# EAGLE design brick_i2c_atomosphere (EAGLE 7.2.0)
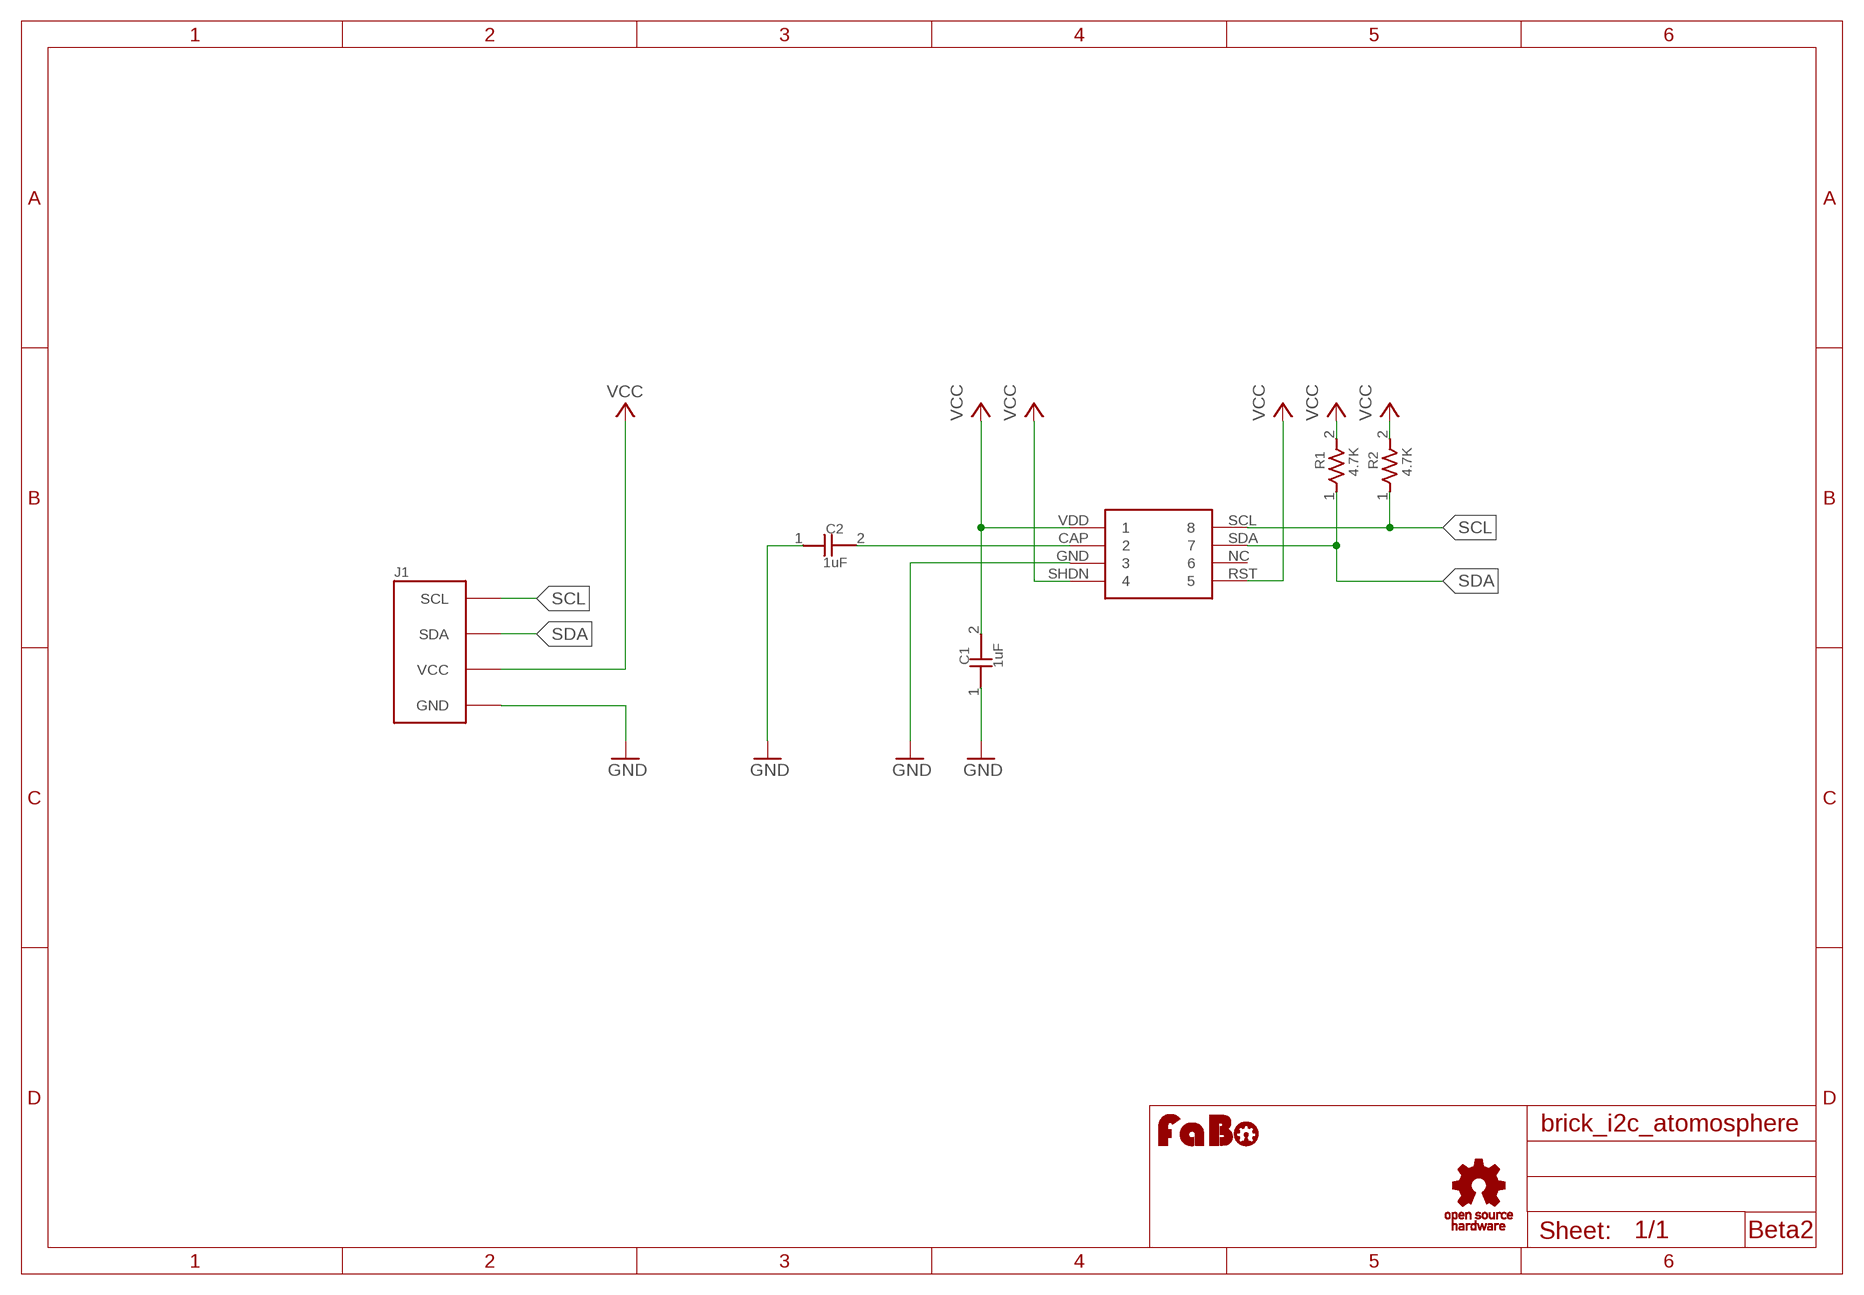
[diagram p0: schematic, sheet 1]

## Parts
C1  1uF  CAPACITOR0603  [0603]
C2  1uF  CAPACITOR0603  [0603]
J1  BRICK_I2C  [BRICK_I2C]
R1  4.7K  RESISTOR0603  [0603]
R2  4.7K  RESISTOR0603  [0603]
U$2  I2C-MPL115A2  [I2C-MLP115A2]
U$3  LOGO_FABO-M  [LOGO_FABO_M]
U$5  LOGO_OSHW_T-M  [LOGO_OSHW_T_M]

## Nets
GND: C1.1 C2.1 J1.GND U$2.GND
N$1: C2.2 U$2.CAP
SCL: J1.SCL R2.1 U$2.SCL
SDA: J1.SDA R1.1 U$2.SDA
VCC: C1.2 J1.VCC R1.2 R2.2 U$2.RST U$2.SHDN U$2.VDD
Unconnected: U$2.NC

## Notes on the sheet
- Beta2

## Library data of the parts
C1 C2 = GClue-Capacitor:CAPACITOR
J1 = gclue:BRICK_I2C: FaBo Brick 4pin(I2C)
R1 R2 = GClue-Resistors:RESISTOR
U$2 = gclue:I2C-MPL115A2
U$3 = FaBo:LOGO_FABO
U$5 = gclue:LOGO_OSHW_T

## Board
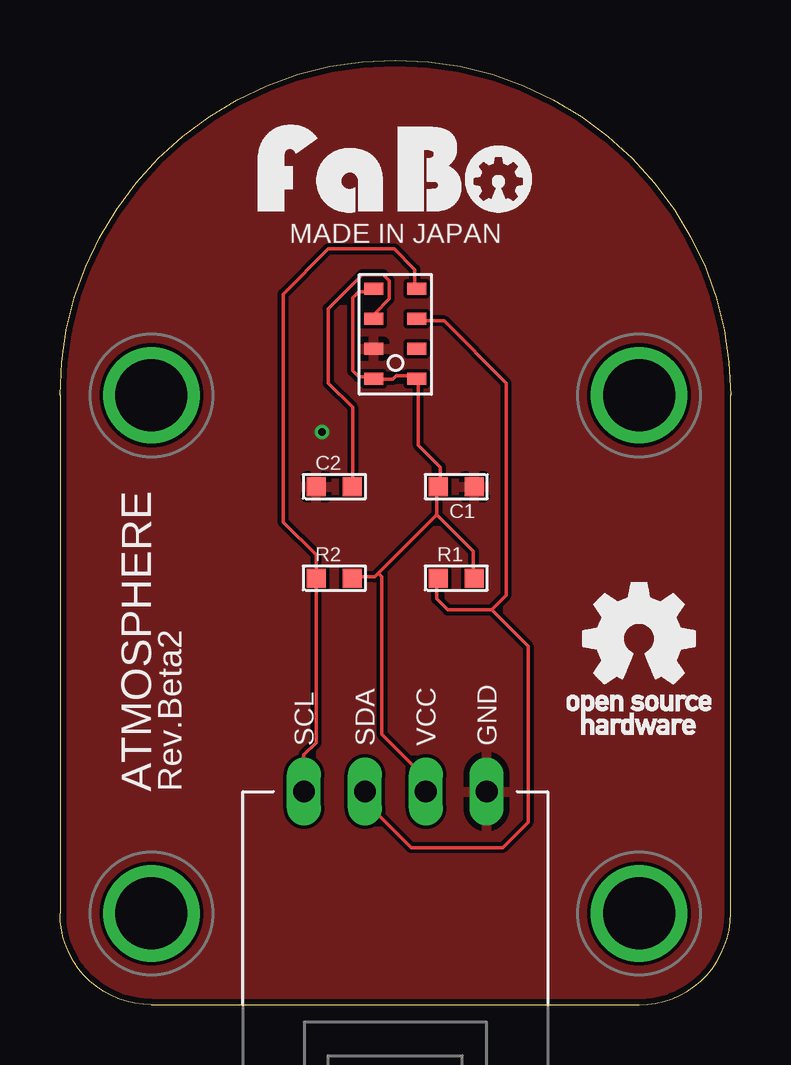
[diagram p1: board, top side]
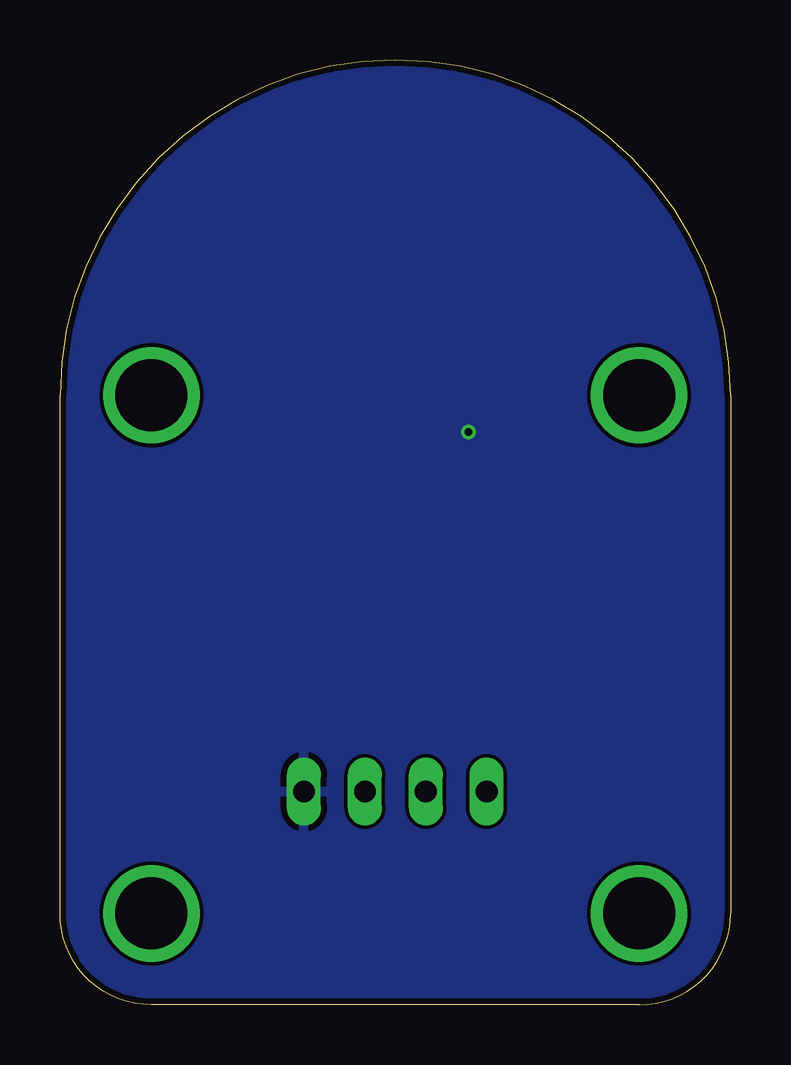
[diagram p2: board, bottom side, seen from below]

Size 27.94 x 39.37 mm. Coordinates in mm from the lower left corner, seen from the top.
Copper layers (1*16): Top 0.035mm / dielectric 1.5mm / Bottom 0.035mm
Design rules "Elecrow_2-layer_eagle_rule": minimum track width 6mil, minimum drill 12mil, track to track 6mil, track to pad 6mil, pad to pad 6mil, via to via 6mil, smd to smd 0mil, copper to edge 10mil, drill to drill 10mil, minimum pad ring 10mil, minimum via ring 6mil, stop-mask expansion 2mil, vias tented up to drill 100mil, thermal gap 10mil

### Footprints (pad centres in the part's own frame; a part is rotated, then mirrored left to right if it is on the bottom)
0603 = smd 0.8 x 0.8: 1 -0.75,0; 2 0.75,0
BRICK_I2C = drill 0.9 long: GND 3.81,-10.16; SCL -3.81,-10.16; SDA -1.27,-10.16; VCC 1.27,-10.16 | drill 3 pad 3.81: P$1 -10.16,6.35; P$2 10.16,6.35; P$3 -10.16,-15.24; P$4 10.16,-15.24
I2C-MLP115A2 = smd 0.8 x 0.5: CAP -0.9,0.65; GND -0.9,-0.6; NC 0.9,-0.6; RST 0.9,-1.85; SCL 0.9,1.9; SDA 0.9,0.65; SHDN -0.9,-1.85; VDD -0.9,1.9

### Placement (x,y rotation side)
C1  16.51,21.59 180 top
C2  11.43,21.59 0 top
J1  13.97,19.05 0 top
R1  16.51,17.78 0 top
R2  11.43,17.78 0 top
U$2  13.97,27.94 0 top
U$3  13.97,33.02 0 top
U$5  24.13,15.24 0 top

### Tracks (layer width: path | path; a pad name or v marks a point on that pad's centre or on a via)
GND  (via drill 0.3)
  other vias: 10.92,23.88
  pour Bottom: -1.27,-1.27 29.21,-1.27 29.21,40.64 -1.27,40.64
  pour Top: -1.27,-1.27 29.21,-1.27 29.21,40.64 -1.27,40.64
N$1
  Top 0.152: C2.2 12.19,21.64 12.19,24.89 11.18,25.91 11.18,29.01 12.6,30.43 13.46,30.43 13.72,30.18 13.72,29.41 13.11,28.8 13.26,28.65 13.11,28.5 U$2.CAP
SCL
  Top 0.152: J1.SCL 10.16,10.41 10.67,10.92 10.67,17.68 R2.1 10.67,17.83 10.67,18.75 9.3,20.12 9.3,29.62 11.18,31.5 13.92,31.5 14.78,30.63 14.78,29.87 U$2.SCL
SDA
  Top 0.152: 17.98,16.46 18.59,17.07 18.59,25.91 16,28.5 14.94,28.5 U$2.SDA | 17.98,16.46 16.15,16.46 15.7,16.92 15.7,17.68 R1.1 | 17.98,16.46 19.51,14.94 19.51,7.62 18.44,6.55 14.63,6.55 12.8,8.38 12.8,8.84 J1.SDA
VCC
  Top 0.152: U$2.VDD 12.95,29.87 12.9,29.87 12.7,29.72 12.45,29.72 12.19,29.46 12.19,26.42 12.45,26.16 12.95,26.16 U$2.SHDN 13.11,26.06 13.87,26.06 14.02,26.21 14.78,26.21 U$2.RST 14.94,26.06 14.94,23.32 15.85,22.4 15.85,21.64 C1.2 15.7,21.49 15.7,20.42 | 15.7,20.42 13.26,17.98 | 13.26,17.98 13.11,17.83 12.19,17.83 R2.2 | 15.7,20.42 17.22,18.9 17.22,17.83 R1.2 | J1.VCC 15.24,9.45 13.41,11.28 13.41,17.83 13.26,17.98

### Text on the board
tPlace: MADE IN JAPAN | ATMOSPHERE | Rev.Beta2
